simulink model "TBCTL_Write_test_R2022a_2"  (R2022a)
settings: Solver=FixedStepDiscrete  StartTime=0.0  StopTime=inf  RelTol=1e-3  EnableMultiTasking=on
InitFcn:
  | Frequency = 800;
  | PeriodPWM = 1/Frequency / 2 * 100e6;
  | Tcontrol = 5e-5;
  | TcontrolInv = 2e-4;
model workspace (MAT data in the model file):
  VoRef = 700
undefined symbols (not defined in the file): A, After, Before, bin2dec, Code, Compare, conversion, Custom, DCAEVT1, DCAEVT1FILT, Digital, Down, EALLOW, EDIS, Event, Filtered, GPTRIP1SEL, GPTRIP2SEL, hex2dec, input, Module, of, start, Trip, TZ1, TZ2, Up, version, Write, Zone
libraries: idelinklib_common x6, c2837xDlib x3, simulink x2, c2802xlib x2

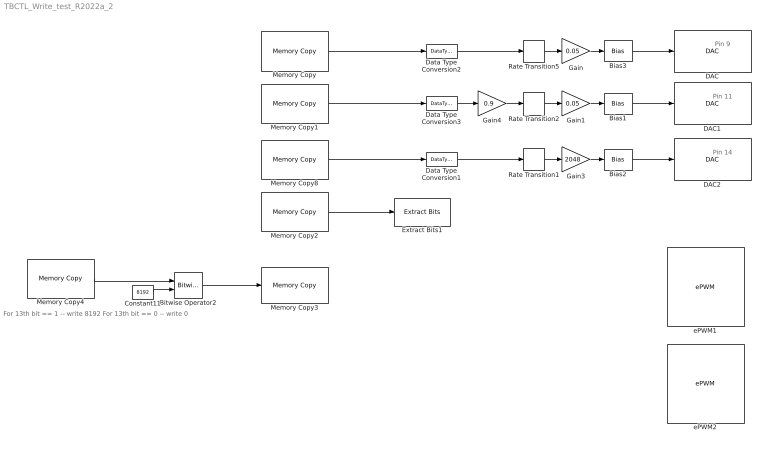
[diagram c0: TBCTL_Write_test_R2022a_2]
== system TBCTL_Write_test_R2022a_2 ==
  note: Pin 11
  note: Pin 14
  note: Pin 9
  note: For 13th bit == 1 -- write 8192 For 13th bit == 0 -- write 0
  Bias1 : Bias
  Bias2 : Bias
  Bias3 : Bias
  Bitwise Operator2 : simulink/Logic and Bit Operations/Bitwise Operator  logicop=XOR  UseBitMask=off  NumInputPorts=2  BitMask=bin2dec('11011001')  BitMaskRealWorld=Stored Integer
  Constant11 : Constant  Value=8192  OutDataTypeStr=uint32
  DAC : c2837xDlib/DAC  channel=A  saturate=off
  DAC1 : c2837xDlib/DAC  channel=B  saturate=off
  DAC2 : c2837xDlib/DAC  channel=C  saturate=off
  Data Type Conversion1 : DataTypeConversion  OutDataTypeStr=single
  Data Type Conversion2 : DataTypeConversion  OutDataTypeStr=single
  Data Type Conversion3 : DataTypeConversion  OutDataTypeStr=single
  Extract Bits1 : simulink/Logic and Bit Operations/Extract Bits  Commented=on  bitsToExtract=Range of bits  numBits=3  bitIdxRange=[13]  outScalingMode=Treat bit field as an integer
  Gain : Gain  Gain=0.05
  Gain1 : Gain  Gain=0.05
  Gain3 : Gain  Gain=2048
  Gain4 : Gain  Gain=0.9
  Memory Copy : idelinklib_common/Memory Copy  copyFrom=Specified source code symbol  copyFromAddressSource=Specify via dialog  copyFromAddress=hex2dec('00001000')  copyFromSrcCode=&EPwm1Regs.TBCTR  dataTypeFrom=uint16  dataDimensionFrom=1  useOffsetFrom=off  offsetFromSrc=Input port  offsetFrom=0  strideFrom=1  copyTo=Output port  copyToAddressSource=Input port  copyToAddress=hex2dec('00002000')  copyToSrcCode=myVariableDst  dataTypeTo=uint32  useOffsetTo=off  offsetToSrc=Specify via dialog  offsetTo=0  strideTo=1  sampleTime=Tcontrol  useInitValue=off  initValueSrc=Specify constant value  initValue=1  initValueSrcCode=myInitValueVariable  useAsMask=off  maskOperator=bitwise AND  useTermValue=off  termValue=1  isRealtimeEnabled=off  emitCCBeforeWrite=off  CCBeforeWrite=/* Custom Code Before Write*/  emitCCAfterWrite=off  CCAfterWrite=/* Custom Code After Write*/  useDMACopy=off  enableBlockingMode=off
  Memory Copy1 : idelinklib_common/Memory Copy  copyFrom=Specified source code symbol  copyFromAddressSource=Specify via dialog  copyFromAddress=hex2dec('00001000')  copyFromSrcCode=&EPwm2Regs.TBCTR  dataTypeFrom=uint16  dataDimensionFrom=1  useOffsetFrom=off  offsetFromSrc=Input port  offsetFrom=0  strideFrom=1  copyTo=Output port  copyToAddressSource=Input port  copyToAddress=hex2dec('00002000')  copyToSrcCode=myVariableDst  dataTypeTo=uint32  useOffsetTo=off  offsetToSrc=Specify via dialog  offsetTo=0  strideTo=1  sampleTime=Tcontrol  useInitValue=off  initValueSrc=Specify constant value  initValue=1  initValueSrcCode=myInitValueVariable  useAsMask=off  maskOperator=bitwise AND  useTermValue=off  termValue=1  isRealtimeEnabled=off  emitCCBeforeWrite=off  CCBeforeWrite=/* Custom Code Before Write*/  emitCCAfterWrite=off  CCAfterWrite=/* Custom Code After Write*/  useDMACopy=off  enableBlockingMode=off
  Memory Copy2 : idelinklib_common/Memory Copy  Commented=on  copyFrom=Specified source code symbol  copyFromAddressSource=Specify via dialog  copyFromAddress=hex2dec('00001000')  copyFromSrcCode=&EPwm2Regs.TBCTL  dataTypeFrom=uint32  dataDimensionFrom=1  useOffsetFrom=off  offsetFromSrc=Input port  offsetFrom=0  strideFrom=1  copyTo=Output port  copyToAddressSource=Input port  copyToAddress=hex2dec('00002000')  copyToSrcCode=myVariableDst  dataTypeTo=uint32  useOffsetTo=off  offsetToSrc=Specify via dialog  offsetTo=0  strideTo=1  sampleTime=Tcontrol  useInitValue=off  initValueSrc=Specify constant value  initValue=1  initValueSrcCode=myInitValueVariable  useAsMask=off  maskOperator=bitwise AND  useTermValue=off  termValue=1  isRealtimeEnabled=off  emitCCBeforeWrite=off  CCBeforeWrite=/* Custom Code Before Write*/  emitCCAfterWrite=off  CCAfterWrite=/* Custom Code After Write*/  useDMACopy=off  enableBlockingMode=off
  Memory Copy3 : idelinklib_common/Memory Copy  copyFrom=Input port  copyFromAddressSource=Specify via dialog  copyFromAddress=hex2dec('00001000')  copyFromSrcCode=myVariableSrc  dataTypeFrom=uint32  dataDimensionFrom=1  useOffsetFrom=off  offsetFromSrc=Specify via dialog  offsetFrom=0  strideFrom=1  copyTo=Specified source code symbol  copyToAddressSource=Specify via dialog  copyToAddress=hex2dec('00002000')  copyToSrcCode=EPwm2Regs.TBPRD  dataTypeTo=uint32  useOffsetTo=off  offsetToSrc=Specify via dialog  offsetTo=0  strideTo=1  sampleTime=inf  useInitValue=off  initValueSrc=Specify constant value  initValue=1  initValueSrcCode=myInitValueVariable  useAsMask=off  maskOperator=bitwise AND  useTermValue=off  termValue=1  isRealtimeEnabled=off  emitCCBeforeWrite=on  CCBeforeWrite=EALLOW;  emitCCAfterWrite=on  CCAfterWrite=EDIS;  useDMACopy=off  enableBlockingMode=off
  Memory Copy4 : idelinklib_common/Memory Copy  copyFrom=Specified source code symbol  copyFromAddressSource=Specify via dialog  copyFromAddress=hex2dec('00001000')  copyFromSrcCode=&EPwm2Regs.TBCTL  dataTypeFrom=uint32  dataDimensionFrom=1  useOffsetFrom=off  offsetFromSrc=Input port  offsetFrom=0  strideFrom=1  copyTo=Output port  copyToAddressSource=Input port  copyToAddress=hex2dec('00002000')  copyToSrcCode=myVariableDst  dataTypeTo=uint32  useOffsetTo=off  offsetToSrc=Specify via dialog  offsetTo=0  strideTo=1  sampleTime=Tcontrol  useInitValue=off  initValueSrc=Specify constant value  initValue=1  initValueSrcCode=myInitValueVariable  useAsMask=off  maskOperator=bitwise AND  useTermValue=off  termValue=1  isRealtimeEnabled=off  emitCCBeforeWrite=off  CCBeforeWrite=/* Custom Code Before Write*/  emitCCAfterWrite=off  CCAfterWrite=/* Custom Code After Write*/  useDMACopy=off  enableBlockingMode=off
  Memory Copy8 : idelinklib_common/Memory Copy  copyFrom=Specified source code symbol  copyFromAddressSource=Specify via dialog  copyFromAddress=hex2dec('00001000')  copyFromSrcCode=&EPwm2Regs.TBCTL.bit.PHSDIR  dataTypeFrom=boolean  dataDimensionFrom=1  useOffsetFrom=off  offsetFromSrc=Input port  offsetFrom=0  strideFrom=1  copyTo=Output port  copyToAddressSource=Input port  copyToAddress=hex2dec('00002000')  copyToSrcCode=myVariableDst  dataTypeTo=boolean  useOffsetTo=off  offsetToSrc=Specify via dialog  offsetTo=0  strideTo=1  sampleTime=Tcontrol  useInitValue=off  initValueSrc=Specify constant value  initValue=1  initValueSrcCode=myInitValueVariable  useAsMask=off  maskOperator=bitwise AND  useTermValue=off  termValue=1  isRealtimeEnabled=off  emitCCBeforeWrite=off  CCBeforeWrite=/* Custom Code Before Write*/  emitCCAfterWrite=off  CCAfterWrite=/* Custom Code After Write*/  useDMACopy=off  enableBlockingMode=off
  Rate Transition1 : RateTransition  OutPortSampleTime=TcontrolInv
  Rate Transition2 : RateTransition  OutPortSampleTime=Tcontrol
  Rate Transition5 : RateTransition  OutPortSampleTime=Tcontrol
  ePWM1 : c2802xlib/ePWM  PwmType=C2000_Type4  useModule=ePWM1  ePWMxLINKTBPRD=Not Linked  periodUnits=Clock cycles  timerSource=Specify via dialog  timerPeriod_clk=PeriodPWM  timerPeriod_sec=0.0001  tbshadow=Counter equals to zero  countingMode=Up-Down  phaseActiveEnable=Disable  phaseDirection=Count up after sync  phaseActive=0  synchronizationEnable=off  dcaevt1Sync=off  dcbevt1Sync=off  synchronizationOption=Counter equals to zero (CTR=Zero)  perSynchronizationOption=Counter equals to period (CTR=PRD)  clockPrescale=1  HSclockPrescale=1  enswap=off  ePWMxAStatus=on  ePWMxAactionLogic1=Set  ePWMxAactionLogic2=Clear  ePWMxAactionLogic3=Clear  ePWMxAactionLogic4=Set  ePWMxAactionLogic5=Do nothing  ePWMxAactionLogic6=Do nothing  ePWMxACSFenable=off  ePWMxACSFvalue=Forcing disable  ePWMxASFreload=Zero  ePWMxBStatus=on  ePWMxBactionLogic1=Clear  ePWMxBactionLogic2=Set  ePWMxBactionLogic3=Do nothing  ePWMxBactionLogic4=Do nothing  ePWMxBactionLogic5=Set  ePWMxBactionLogic6=Clear  ePWMxBCSFenable=off  ePWMxBCSFvalue=Forcing disable  ePWMxBSFreload=Zero  ePWNxBOutWay=off  ePWMxLINKCMPA=Not Linked  CMPAUnits=Clock cycles  CMPASource=Specify via dialog  CMPAValue_per=50  CMPAValue_clk=PeriodPWM  enCMPAshadow=Counter equals to zero (CTR=Zero)  ePWMxLINKCMPB=Not Linked  CMPBUnits=Clock cycles  CMPBSource=Specify via dialog  CMPBValue_per=50  CMPBValue_clk=PeriodPWM  enCMPBshadow=Counter equals to zero (CTR=Zero)  ePWMxLINKCMPC=Not Linked  CMPCUnits=Clock cycles  CMPCSource=Specify via dialog  CMPCValue_per=50  CMPCValue_clk=32000  enCMPCshadow=Counter equals to zero (CTR=Zero)  ePWMxLINKCMPD=Not Linked  CMPDUnits=Clock cycles  CMPDSource=Specify via dialog  CMPDValue_per=50  CMPDValue_clk=32000  enCMPDshadow=Counter equals to zero (CTR=Zero)  enableDBePWMxA=off  enableDBePWMxB=off  enhalfcycle=off  DBpolarity=Active high complementary (AHC)  DBedgeDelay=Positive  DBSource_ePWMxA=ePWMxA  DBSource_ePWMxB=ePWMxA  DBPeriodUnits=Clock cycles  DBperiodSource=Input port  REDperiod=0  FEDperiod=0  REDperiod_sec=0  FEDperiod_sec=0  LoadModeDBRED=Immediate without using shadow  LoadModeDBFED=Immediate without using shadow  adcstartModuleA=off  adcrequestEventA=First event  adcstartEventA=Digital Compare Module A Event 1 start of conversion (DCAEVT1.soc)  adcstartEventA_type2=Digital Compare Module A Event 1 start of conversion (DCAEVT1.soc)  adcstartModuleB=off  adcrequestEventB=First event  adcstartEventB=Counter equals to zero (CTR=Zero)  adcstartEventB_type2=Counter equals to zero (CTR=Zero)  intEn=on  intPrd=First event  intSel=Counter equals to zero (CTR=Zero)  intSel_type2=Counter equals to zero (CTR=Zero)  hrpe=off  enHRPWM=off  HRPWM_LoadMode=Counter equals to period (CTR=PRD)  HRPWM_CTLMode=Duty or Period control mode  HRPWM_EDGMode=Both edge  hrpeb=off  enHRPWMB=off  HRPWM_LoadModeB=Counter equals to zero (CTR=ZERO)  HRPWM_CTLModeB=Duty or Period control mode  HRPWM_EDGModeB=Both edge  enHRDBRED=off  enHRDBFED=off  enSFO=on  enautoconv=on  chopperEnable=off  chopperFrequency=1  chopperFirstwidth=1  chopperDuty=12.5%  tripZonesource=Specify via dialog  tzselOSHT1=off  tzselOSHT2=off  tzselOSHT3=off  tzselOSHDCAEV1=off  tzselOSHDCBEV1=off  tzselCBC1=off  tzselCBC2=off  tzselCBC3=off  tzselCBCDCAEV2=off  tzselCBCDCBEV2=off  tzselOSHT4=off  tzselOSHT5=off  tzselOSHT6=off  tzselCBC4=off  tzselCBC5=off  tzselCBC6=off  enTzOstIntr=off  enTzCbcIntr=off  enTzDCAEVT1Intr=off  enTzDCAEVT2Intr=off  enTzDCBEVT1Intr=off  enTzDCBEVT2Intr=off  ePWMxAforced=No action  ePWMxBforced=No action  DCAEVT1forced=No action  DCBEVT1forced=No action  DCAEVT2forced=No action  DCBEVT2forced=No action  dcah=Trip Zone 1 input (TZ1)  dcal=Trip Zone 2 input (TZ2)  dcbh=Trip Zone 1 input (TZ1)  dcbl=Trip Zone 2 input (TZ2)  dcah_type2=GPTRIP1SEL/(TZ1)  dcal_type2=GPTRIP2SEL/(TZ2)  dcbh_type2=GPTRIP1SEL/(TZ1)  dcbl_type2=GPTRIP2SEL/(TZ2)  gendcaevt1=Event disabled  gendcaevt2=Event disabled  gendcbevt1=Event disabled  gendcbevt2=Event disabled  dcaevt1src=DCAEVT1 with sync  dcaevt2src=DCAEVT2 with sync  dcbevt1src=DCBEVT1 with sync  dcbevt2src=DCBEVT2 with sync  pulsesel=Counter equals to zero (CTR=Zero)  blankinv=off  blankoffset=0  blankwidth=0  evsrcsel=Filtered version of DCAEVT1 (DCAEVT1FILT)  encape=off
  ePWM2 : c2802xlib/ePWM  PwmType=C2000_Type4  useModule=ePWM2  ePWMxLINKTBPRD=Not Linked  periodUnits=Clock cycles  timerSource=Specify via dialog  timerPeriod_clk=PeriodPWM  timerPeriod_sec=0.0001  tbshadow=Counter equals to zero  countingMode=Up-Down  phaseActiveEnable=Disable  phaseDirection=Count down after sync  phaseActive=PeriodPWM  synchronizationEnable=off  dcaevt1Sync=off  dcbevt1Sync=off  synchronizationOption=Counter equals to zero (CTR=Zero)  perSynchronizationOption=Counter equals to period (CTR=PRD)  clockPrescale=1  HSclockPrescale=1  enswap=off  ePWMxAStatus=on  ePWMxAactionLogic1=Set  ePWMxAactionLogic2=Clear  ePWMxAactionLogic3=Clear  ePWMxAactionLogic4=Set  ePWMxAactionLogic5=Do nothing  ePWMxAactionLogic6=Do nothing  ePWMxACSFenable=off  ePWMxACSFvalue=Forcing disable  ePWMxASFreload=Zero  ePWMxBStatus=on  ePWMxBactionLogic1=Clear  ePWMxBactionLogic2=Set  ePWMxBactionLogic3=Do nothing  ePWMxBactionLogic4=Do nothing  ePWMxBactionLogic5=Set  ePWMxBactionLogic6=Clear  ePWMxBCSFenable=off  ePWMxBCSFvalue=Forcing disable  ePWMxBSFreload=Zero  ePWNxBOutWay=off  ePWMxLINKCMPA=Not Linked  CMPAUnits=Clock cycles  CMPASource=Specify via dialog  CMPAValue_per=50  CMPAValue_clk=3750  enCMPAshadow=Counter equals to zero (CTR=Zero)  ePWMxLINKCMPB=Not Linked  CMPBUnits=Clock cycles  CMPBSource=Specify via dialog  CMPBValue_per=50  CMPBValue_clk=3750  enCMPBshadow=Counter equals to zero (CTR=Zero)  ePWMxLINKCMPC=Not Linked  CMPCUnits=Clock cycles  CMPCSource=Specify via dialog  CMPCValue_per=50  CMPCValue_clk=32000  enCMPCshadow=Counter equals to zero (CTR=Zero)  ePWMxLINKCMPD=Not Linked  CMPDUnits=Clock cycles  CMPDSource=Specify via dialog  CMPDValue_per=50  CMPDValue_clk=32000  enCMPDshadow=Counter equals to zero (CTR=Zero)  enableDBePWMxA=off  enableDBePWMxB=off  enhalfcycle=off  DBpolarity=Active high complementary (AHC)  DBedgeDelay=Positive  DBSource_ePWMxA=ePWMxA  DBSource_ePWMxB=ePWMxA  DBPeriodUnits=Clock cycles  DBperiodSource=Input port  REDperiod=0  FEDperiod=0  REDperiod_sec=0  FEDperiod_sec=0  LoadModeDBRED=Immediate without using shadow  LoadModeDBFED=Immediate without using shadow  adcstartModuleA=off  adcrequestEventA=First event  adcstartEventA=Digital Compare Module A Event 1 start of conversion (DCAEVT1.soc)  adcstartEventA_type2=Digital Compare Module A Event 1 start of conversion (DCAEVT1.soc)  adcstartModuleB=off  adcrequestEventB=First event  adcstartEventB=Counter equals to zero (CTR=Zero)  adcstartEventB_type2=Counter equals to zero (CTR=Zero)  intEn=off  intPrd=First event  intSel=Counter equals to zero (CTR=Zero)  intSel_type2=Counter equals to zero (CTR=Zero)  hrpe=off  enHRPWM=off  HRPWM_LoadMode=Counter equals to period (CTR=PRD)  HRPWM_CTLMode=Duty or Period control mode  HRPWM_EDGMode=Both edge  hrpeb=off  enHRPWMB=off  HRPWM_LoadModeB=Counter equals to zero (CTR=ZERO)  HRPWM_CTLModeB=Duty or Period control mode  HRPWM_EDGModeB=Both edge  enHRDBRED=off  enHRDBFED=off  enSFO=on  enautoconv=on  chopperEnable=off  chopperFrequency=1  chopperFirstwidth=1  chopperDuty=12.5%  tripZonesource=Specify via dialog  tzselOSHT1=off  tzselOSHT2=off  tzselOSHT3=off  tzselOSHDCAEV1=off  tzselOSHDCBEV1=off  tzselCBC1=off  tzselCBC2=off  tzselCBC3=off  tzselCBCDCAEV2=off  tzselCBCDCBEV2=off  tzselOSHT4=off  tzselOSHT5=off  tzselOSHT6=off  tzselCBC4=off  tzselCBC5=off  tzselCBC6=off  enTzOstIntr=off  enTzCbcIntr=off  enTzDCAEVT1Intr=off  enTzDCAEVT2Intr=off  enTzDCBEVT1Intr=off  enTzDCBEVT2Intr=off  ePWMxAforced=No action  ePWMxBforced=No action  DCAEVT1forced=No action  DCBEVT1forced=No action  DCAEVT2forced=No action  DCBEVT2forced=No action  dcah=Trip Zone 1 input (TZ1)  dcal=Trip Zone 2 input (TZ2)  dcbh=Trip Zone 1 input (TZ1)  dcbl=Trip Zone 2 input (TZ2)  dcah_type2=GPTRIP1SEL/(TZ1)  dcal_type2=GPTRIP2SEL/(TZ2)  dcbh_type2=GPTRIP1SEL/(TZ1)  dcbl_type2=GPTRIP2SEL/(TZ2)  gendcaevt1=Event disabled  gendcaevt2=Event disabled  gendcbevt1=Event disabled  gendcbevt2=Event disabled  dcaevt1src=DCAEVT1 with sync  dcaevt2src=DCAEVT2 with sync  dcbevt1src=DCBEVT1 with sync  dcbevt2src=DCBEVT2 with sync  pulsesel=Counter equals to zero (CTR=Zero)  blankinv=off  blankoffset=0  blankwidth=0  evsrcsel=Filtered version of DCAEVT1 (DCAEVT1FILT)  encape=off
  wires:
  Rate Transition2/1 -> Gain1/1
  Data Type Conversion1/1 -> Rate Transition1/1
  Data Type Conversion3/1 -> Gain4/1
  Rate Transition1/1 -> Gain3/1
  Rate Transition5/1 -> Gain/1
  Gain/1 -> Bias3/1
  Bias1/1 -> DAC1/1
  Gain3/1 -> Bias2/1
  Gain1/1 -> Bias1/1
  Bias3/1 -> DAC/1
  Data Type Conversion2/1 -> Rate Transition5/1
  Memory Copy/1 -> Data Type Conversion2/1
  Memory Copy1/1 -> Data Type Conversion3/1
  Gain4/1 -> Rate Transition2/1
  Memory Copy8/1 -> Data Type Conversion1/1
  Memory Copy2/1 -> Extract Bits1/1
  Bitwise Operator2/1 -> Memory Copy3/1
  Constant11/1 -> Bitwise Operator2/2
  Memory Copy4/1 -> Bitwise Operator2/1
  Bias2/1 -> DAC2/1
